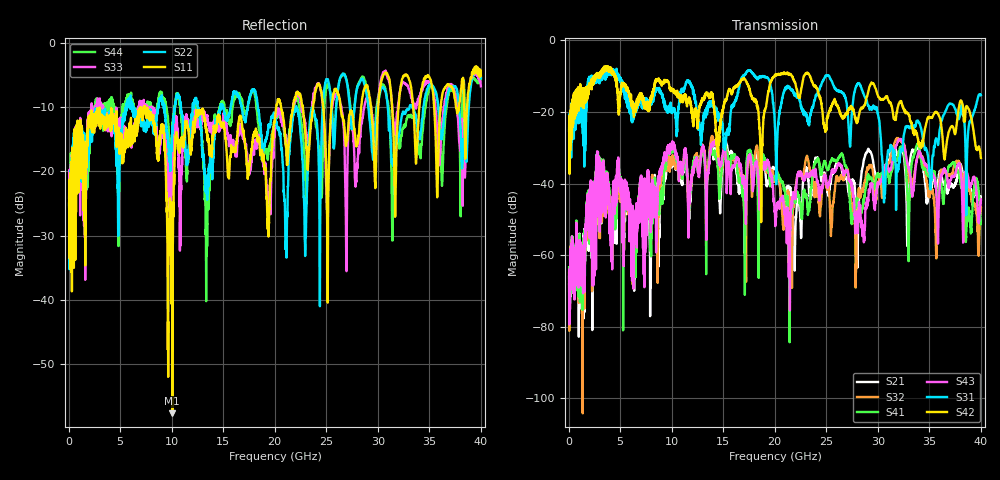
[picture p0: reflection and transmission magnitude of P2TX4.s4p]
!Agilent Technologies,N5245A,MY49151084,A.09.20.08
!Agilent N5245A: A.09.20.08
!Date: Thursday, March 01, 2012 12:03:37
!Correction: S11(Full 4 Port(1,2,3,4))
!S12(Full 4 Port(1,2,3,4))
!S13(Full 4 Port(1,2,3,4))
!S14(Full 4 Port(1,2,3,4))
!S21(Full 4 Port(1,2,3,4))
!S22(Full 4 Port(1,2,3,4))
!S23(Full 4 Port(1,2,3,4))
!S24(Full 4 Port(1,2,3,4))
!S31(Full 4 Port(1,2,3,4))
!S32(Full 4 Port(1,2,3,4))
!S33(Full 4 Port(1,2,3,4))
!S34(Full 4 Port(1,2,3,4))
!S41(Full 4 Port(1,2,3,4))
!S42(Full 4 Port(1,2,3,4))
!S43(Full 4 Port(1,2,3,4))
!S44(Full 4 Port(1,2,3,4))
!S4P File: Measurements: <S11,S12,S13,S14>,
!<S21,S22,S23,S24>,
!<S31,S32,S33,S34>,
!<S41,S42,S43,S44>:
# Hz S  dB  R 50
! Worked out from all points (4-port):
!   3996 points, 50 MHz to 40 GHz, reference 50 ohm
!   strongest paths, dB at 50 MHz, 10.04 GHz, 20.03 GHz, 30.02 GHz, 40 GHz:
!     S42: -25.3, -13.9, -9.7, -15.5, -32.9
!     S31: -24.8, -20.3, -24.6, -20.7, -15.3
!     S43: -68.1, -29.0, -49.2, -40.1, -44.5
!     S41: -63.4, -30.0, -38.4, -37.2, -50.5
!     S32: -65.0, -33.7, -38.9, -40.1, -46.6
!     S21: -66.1, -34.4, -35.7, -37.6, -44.5
!   lowest |S11| = -57.7 dB at 10.06 GHz (marker M1), VSWR 1.00, Z = 49.9 + j0.097 ohm
!   |S11| at or under -10 dB: start of sweep to 7.319 GHz; 7.393 GHz to 20.15 GHz (12.76 GHz wide, 92.6 % of centre); 26.38 GHz to 28.39 GHz (2.017 GHz wide, 7.37 % of centre)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
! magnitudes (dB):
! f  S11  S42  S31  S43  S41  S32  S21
! 50 MHz  -24.9  -25.3  -24.8  -68.1  -63.4  -65.0  -66.1
! 2.89 GHz  -11.0  -10.3  -10.4  -32.6  -33.1  -35.2  -36.2
! 6.45 GHz  -12.6  -18.2  -20.0  -51.7  -59.9  -64.5  -63.3
! 10.06 GHz  -57.7  -13.7  -19.6  -29.4  -30.0  -33.2  -33.9
! 28.16 GHz  -14.3  -20.9  -11.9  -45.7  -45.7  -41.3  -45.3
! 30.66 GHz  -4.7  -16.2  -42.7  -35.7  -35.5  -38.0  -36.9
! 40 GHz  -5.1  -32.9  -15.3  -44.5  -50.5  -46.6  -44.5
